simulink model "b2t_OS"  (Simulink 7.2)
settings: Solver=ode3  SolverMode=SingleTasking  StartTime=0.0  StopTime=0.2  FixedStep=10e-6  MaxStep=1e-5  RelTol=1e-4  AbsTol=1e-4

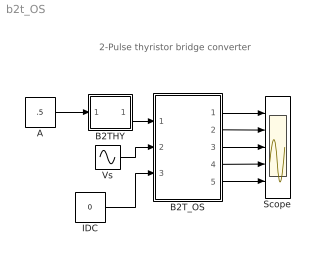
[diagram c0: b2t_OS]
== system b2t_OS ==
  note: 2-Pulse thyristor bridge converter
  A : Constant  Value=.5
  B2THY : Subsystem  mask(M1THY-Con){F=50, PH=90, TD=5e-3}
      mask prompts: F "Frequency"; PH "Phase Angle (Degree)"; TD "Puls Duration"
      mask help: Control of one Thyristor in a line commutated Converter circuit
      mask init:
      | x=0:pi/20:2*pi;
      | y=cos(x);
  B2T_OS : Subsystem  mask{LS=1e-4, LD=10e-3, ILD0=0, C=20e-3, VC0=100, RL=1}
      mask prompts: LS "Source Inductance"; LD "DC Inductance"; ILD0 "Initial current ILD0"; C "Load Cap"; VC0 "Initial Cap Voltage"; RL "Load Resistance"
      mask help: 2-Pulse Thyristor Bridge Converter Input Vector u: u[0]= H1.gate,H4.gate u[1]= H2.gate,H3.gate u[2]= Vs.v u[3]= IDC.i Output Vector y: y[0]= T1.I y[1]= T1.V y[2]= Lc.I y[3]= Ld.I y[4]= VDC.V y[5]= VC.V Parameter Vector p: p[0]= Lc.L p[1]= Ld.L p[2]= Ld.IL0 p[3]= C1.C p[4]= C1.vC0 p[5]= R1.r You can pause the simulation during running, change the Parameters you want and continue the Simulation
  IDC : Constant  Value=0
  Scope : Scope  NumInputPorts=5
  Vs : Sin  Amplitude=230*sqrt(2)  Frequency=50*2*pi  SampleTime=0
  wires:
  A/1 -> B2THY/1(In1)
  B2THY/1(Out1) -> B2T_OS/1(SWs)
  Vs/1 -> B2T_OS/2(vS)
  IDC/1 -> B2T_OS/3(iDC)
  B2T_OS/1(iT1,vT1) -> Scope/1
  B2T_OS/2(Ilc) -> Scope/2
  B2T_OS/3(iLd) -> Scope/3
  B2T_OS/4(vDC) -> Scope/4
  B2T_OS/5(vC) -> Scope/5

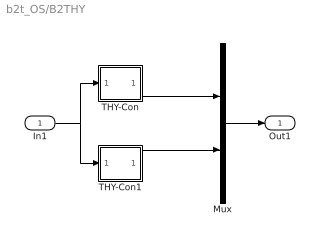
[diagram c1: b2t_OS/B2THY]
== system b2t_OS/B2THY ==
  In1 : Inport
  Mux : Mux  Inputs=2
  THY-Con : Subsystem  mask(THY-Con){F=F, PH=PH, TD=TD}
      mask prompts: F "Frequency"; PH "Phase Angle (Degree)"; TD "Puls Duration"
      mask init:
      | x=0:pi/20:2*pi;
      | y=cos(x);
  THY-Con1 : Subsystem  mask(THY-Con){F=F, PH=-PH, TD=TD}
      mask prompts: F "Frequency"; PH "Phase Angle (Degree)"; TD "Puls Duration"
      mask init:
      | x=0:pi/20:2*pi;
      | y=cos(x);
  Out1 : Outport
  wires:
  In1/1 -> THY-Con1/1(In1), THY-Con/1(In1)
  THY-Con/1(Out1) -> Mux/1
  Mux/1 -> Out1/1
  THY-Con1/1(Out1) -> Mux/2

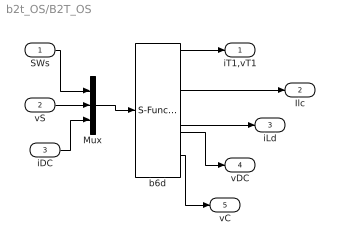
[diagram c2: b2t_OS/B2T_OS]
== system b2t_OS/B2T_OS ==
  SWs : Inport  OutDataType=sfix(16)  OutScaling=2^0
  vS : Inport  Port=2  OutDataType=sfix(16)  OutScaling=2^0
  iDC : Inport  Port=3  OutDataType=sfix(16)  OutScaling=2^0
  Mux : Mux  Inputs="[2 1  1]"
  b6d : S-Function  FunctionName=s_b2t_OS  Parameters="[ LS LD ILD0 C  VC0 RL]"  EnableBusSupport=off
  iT1,vT1 : Outport  OutDataType=sfix(16)  OutScaling=2^0
  Ilc : Outport  Port=2  OutDataType=sfix(16)  OutScaling=2^0
  iLd : Outport  Port=3  OutDataType=sfix(16)  OutScaling=2^0
  vDC : Outport  Port=4  OutDataType=sfix(16)  OutScaling=2^0
  vC : Outport  Port=5  OutDataType=sfix(16)  OutScaling=2^0
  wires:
  b6d/4 -> vDC/1
  Mux/1 -> b6d/1
  iDC/1 -> Mux/3
  b6d/3 -> iLd/1
  b6d/2 -> Ilc/1
  b6d/1 -> iT1,vT1/1
  vS/1 -> Mux/2
  SWs/1 -> Mux/1
  b6d/5 -> vC/1

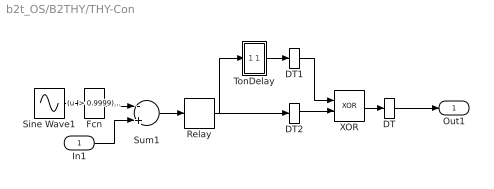
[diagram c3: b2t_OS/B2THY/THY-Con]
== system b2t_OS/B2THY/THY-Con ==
  In1 : Inport
  DT : DataTypeConversion
  DT1 : DataTypeConversion
  DT2 : DataTypeConversion
  Fcn : Fcn  Expr="(u  > 0.9999)*2 + (u<=0.9999)*u"
  Relay : Relay
  Sine Wave1 : Sin  Frequency=F*2*pi  Phase=PH*pi/180  SampleTime=0
  Sum1 : Sum  Inputs=-+
  TonDelay : Subsystem  mask(TonDelay){DT=TD}
      mask prompts: DT "Dead Time"
      mask help: Turn on dead time to protect against short circuit of the converter leg
  XOR : Logic  Operator=XOR
  Out1 : Outport
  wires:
  DT2/1 -> XOR/2
  DT1/1 -> XOR/1
  DT/1 -> Out1/1
  In1/1 -> Sum1/2
  Sum1/1 -> Relay/1
  TonDelay/1(s1d) -> DT1/1
  Relay/1 -> DT2/1, TonDelay/1(s1)
  XOR/1 -> DT/1
  Sine Wave1/1 -> Fcn/1
  Fcn/1 -> Sum1/1

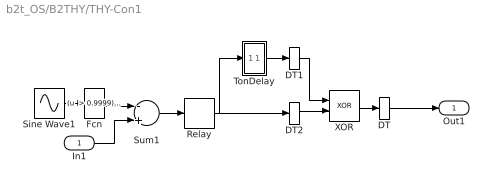
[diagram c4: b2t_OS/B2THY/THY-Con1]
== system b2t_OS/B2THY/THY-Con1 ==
  In1 : Inport
  DT : DataTypeConversion
  DT1 : DataTypeConversion
  DT2 : DataTypeConversion
  Fcn : Fcn  Expr="(u  > 0.9999)*2 + (u<=0.9999)*u"
  Relay : Relay
  Sine Wave1 : Sin  Frequency=F*2*pi  Phase=PH*pi/180  SampleTime=0
  Sum1 : Sum  Inputs=-+
  TonDelay : Subsystem  mask(TonDelay){DT=TD}
      mask prompts: DT "Dead Time"
      mask help: Turn on dead time to protect against short circuit of the converter leg
  XOR : Logic  Operator=XOR
  Out1 : Outport
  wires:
  DT2/1 -> XOR/2
  DT1/1 -> XOR/1
  DT/1 -> Out1/1
  Fcn/1 -> Sum1/1
  Sine Wave1/1 -> Fcn/1
  XOR/1 -> DT/1
  Relay/1 -> DT2/1, TonDelay/1(s1)
  TonDelay/1(s1d) -> DT1/1
  Sum1/1 -> Relay/1
  In1/1 -> Sum1/2

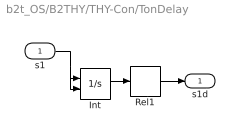
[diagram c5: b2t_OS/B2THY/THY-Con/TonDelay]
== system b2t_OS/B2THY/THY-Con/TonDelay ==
  s1 : Inport
  Int : Integrator  ExternalReset=falling
  Rel1 : Relay  OnSwitchValue=DT
  s1d : Outport  InitialOutput=0
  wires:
  Int/1 -> Rel1/1
  s1/1 -> Int/2, Int/1
  Rel1/1 -> s1d/1

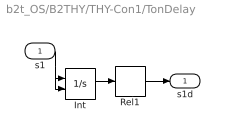
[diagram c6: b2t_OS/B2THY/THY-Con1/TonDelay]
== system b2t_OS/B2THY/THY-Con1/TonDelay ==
  s1 : Inport
  Int : Integrator  ExternalReset=falling
  Rel1 : Relay  OnSwitchValue=DT
  s1d : Outport  InitialOutput=0
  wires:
  Rel1/1 -> s1d/1
  s1/1 -> Int/1, Int/2
  Int/1 -> Rel1/1
